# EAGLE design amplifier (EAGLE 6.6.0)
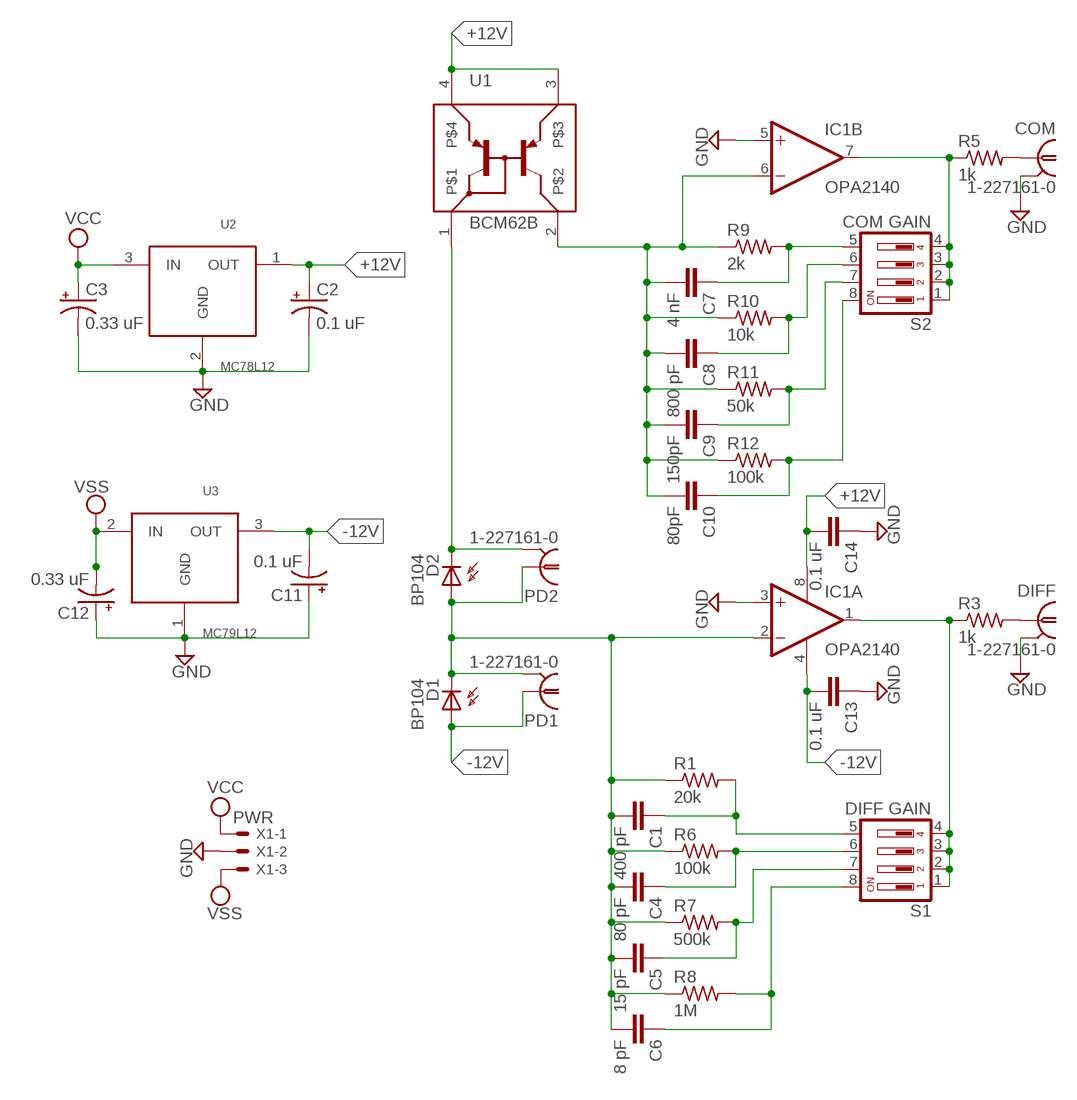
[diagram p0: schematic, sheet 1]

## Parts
C1  400 pF  C-EUC1206K  [C1206K]
C2  0.1 uF  CPOL-USSMCP  [SMC_P]
C3  0.33 uF  CPOL-USSMCP  [SMC_P]
C4  80 pF  C-EUC1206K  [C1206K]
C5  15 pF  C-EUC1206K  [C1206K]
C6  8 pF  C-EUC1206K  [C1206K]
C7  4 nF  C-EUC1206K  [C1206K]
C8  800 pF  C-EUC1206K  [C1206K]
C9  150pF  C-EUC1206K  [C1206K]
C10  80pF  C-EUC1206K  [C1206K]
C11  0.1 uF  CPOL-USSMCP  [SMC_P]
C12  0.33 uF  CPOL-USSMCP  [SMC_P]
C13  0.1 uF  C-EUC1206K  [C1206K]
C14  0.1 uF  C-EUC1206K  [C1206K]
COM  1-227161-0  [AMP_227161]
D1  BP104  [BP104]
D2  BP104  [BP104]
DIFF  1-227161-0  [AMP_227161]
IC1  OPA2140  [SO08]
PD1  1-227161-0  [AMP_227161]
PD2  1-227161-0  [AMP_227161]
R1  20k  R-US_R1206W  [R1206W]
R3  1k  R-US_R1206W  [R1206W]
R5  1k  R-US_R1206W  [R1206W]
R6  100k  R-US_R1206W  [R1206W]
R7  500k  R-US_R1206W  [R1206W]
R8  1M  R-US_R1206W  [R1206W]
R9  2k  R-US_R1206W  [R1206W]
R10  10k  R-US_R1206W  [R1206W]
R11  50k  R-US_R1206W  [R1206W]
R12  100k  R-US_R1206W  [R1206W]
S1  DIFF GAIN  DS04  [DS-04]
S2  COM GAIN  DS04  [DS-04]
U1  BCM62B  [SOT143M]
U2  MC78L12  [TO92-]
U3  MC79L12  [TO92-]
X1  PWR  KK-156-3  [KK-156-3]

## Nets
+12V: C2.+ C14.2 IC1.8(A:V+) U1.3 U1.4 U2.1(OUT)
-12V: C11.- C13.2 D1.A IC1.4(A:V-) PD1.1 U3.3(OUT)
GND: C2.- C3.- C11.+ C12.+ C13.1 C14.1 COM.2 DIFF.2 IC1.3(A:+IN) IC1.5(B:+IN) U2.2(GND) U3.1(GND) X1.2
N$2: C1.1 R1.2 S1.5
N$3: C10.1 R12.2 S2.8
N$5: COM.1 R5.2
N$6: DIFF.1 R3.2
N$8: C1.2 C4.2 C5.2 C6.2 D1.K(C) D2.A IC1.2(A:-IN) PD1.2 PD2.1 R1.1 R6.1 R7.1 R8.1
N$9: D2.K(C) PD2.2 U1.1
N$10: IC1.1(A:OUT) R3.1 S1.1 S1.2 S1.3 S1.4
N$11: C4.1 R6.2 S1.6
N$13: C5.1 R7.2 S1.7
N$14: C6.1 R8.2 S1.8
N$15: IC1.7(B:OUT) R5.1 S2.1 S2.2 S2.3 S2.4
N$16: C9.1 R11.2 S2.7
N$17: C7.1 R9.2 S2.5
N$18: C8.1 R10.2 S2.6
N$20: C7.2 C8.2 C9.2 C10.2 IC1.6(B:-IN) R9.1 R10.1 R11.1 R12.1 U1.2
VCC: C3.+ U2.3(IN) X1.1
VSS: C12.- U3.2(IN) X1.3

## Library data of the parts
C1 C4-C10 C13 C14 = rcl:C-EU: CAPACITOR, European symbol
C2 C3 C11 C12 = rcl:CPOL-US: POLARIZED CAPACITOR, American symbol
COM DIFF PD1 PD2 = con-coax:?227161*: JACK, RIGHT ANGLE, 50 OHM, PCB, BNC; MF: TYCO ELECTRONICS; MPN: 1-227161; OC_FARNELL: unknown; OC_NEWARK: 33B3200
D1 D2 = opto-trans-siemens:BP104: PHOTO DIODE; MF: VISHAY/TELEFUNKEN; MPN: BP104; OC_FARNELL: 1779636; OC_NEWARK: 14M4504
IC1 = Custom parts:OPA2140: Dual Operational Amplifier Low Power, Single-Supply, Rail-To-Rail Operational Amplifier Source: http://focus.ti.com/lit/ds/symlink/opa2345.pdf http://focus.ti.com .. opa241.pdf http://focus.ti.com/lit/ds/symlink/opa2134.pdf
R1 R3 R5-R12 = rcl:R-US_: RESISTOR, American symbol
S1 S2 = switch-dil:DS04: DIL/CODE SWITCH; OC_FARNELL: 9471570; OC_NEWARK: unknown
U1 = Custom parts:BCM62B: BCM61B - PNP/PNP matched double transistor 1.1 General description PNP/PNP matched double transistor in a SOT143B small Surface-Mounted Device (SMD) plastic package. Matched version of BCV62. NPN/NON equivalent: BCM61B 1.2 Features ■ Current gain matching 1.3 Applications ■ Current mirror ■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
U2 = Custom parts:MC78L12: MC78L12 - 100 mA positive +12V voltage resulators The MC78L00A Series of positive voltage regulators are inexpensive, easy–to–use devices suitable for a multitude of applications that require a regulated supply of up to 100 mA. Like their higher powered MC7800 and MC78M00 Series cousins, these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
U3 = Custom parts:MC79L12: MC79L12 - Negative -12V voltage regulator This series of fixed negative-voltage integrated-circuit voltage regulators is designed for a wide range of applications. These include on-card regulation for elimination of noise and distribution problems associated with single-point regulation. In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
X1 = con-molex:KK-156-3: KK 156 HEADER Source: http://www.molex.com/pdm_docs/sd/026604100_sd.pdf; OC_FARNELL: unknown; OC_NEWARK: unknown

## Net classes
0 default: width 0.508 mm, clearance 0.508 mm

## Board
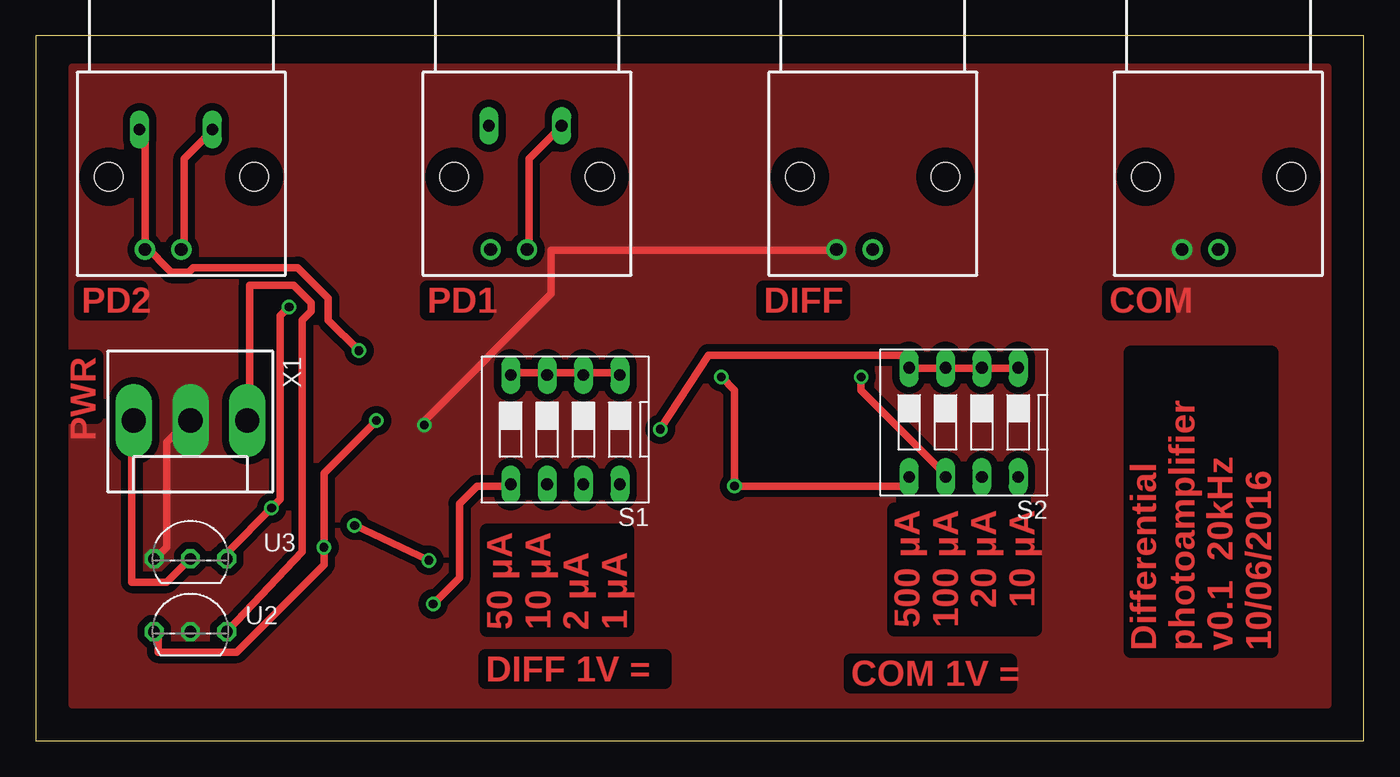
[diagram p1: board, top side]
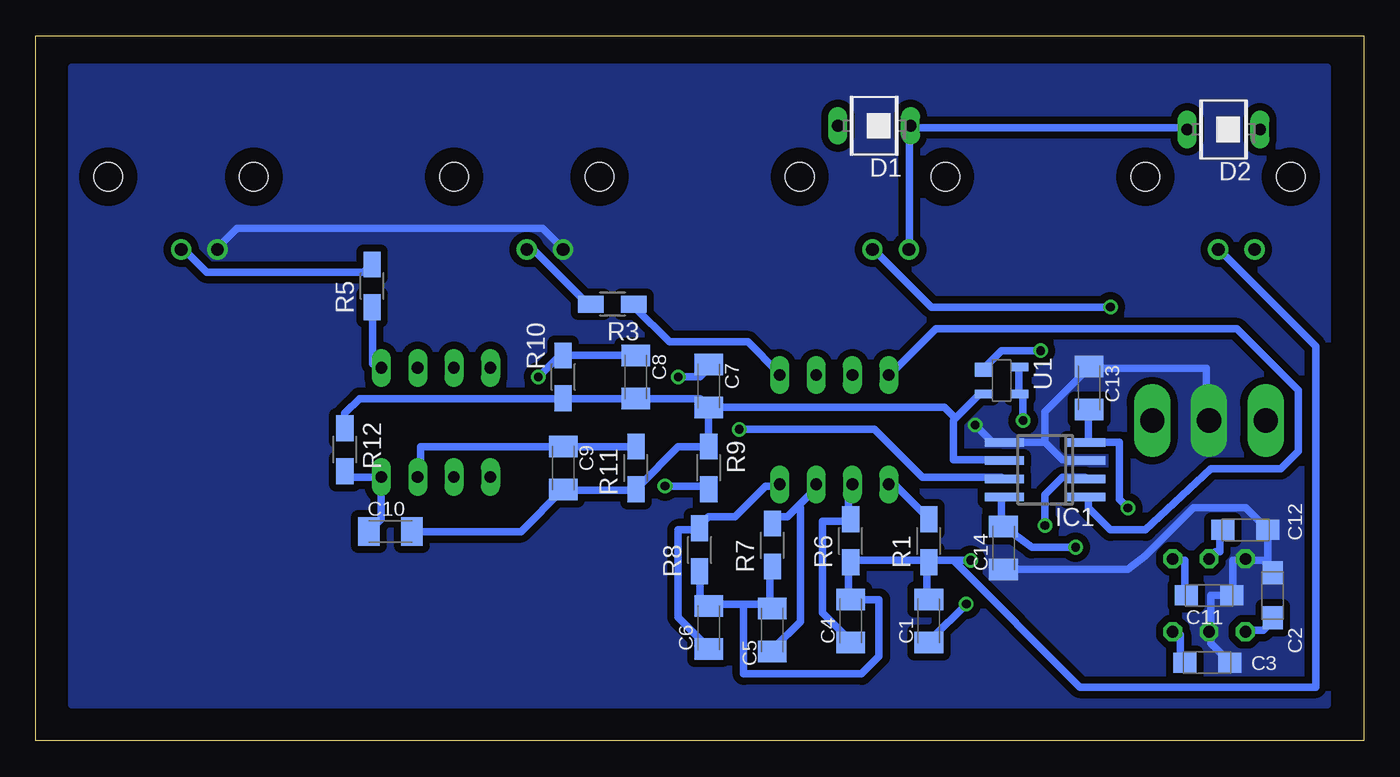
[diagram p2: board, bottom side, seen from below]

Size 92.69 x 49.2 mm. Coordinates in mm from the lower left corner, seen from the top.
Outline: 0,0 92.69,0 92.69,49.2 0,49.2 0,0
Copper layers (1*16): Top 0.035mm / dielectric 1.5mm / Bottom 0.035mm
Design rules "default": minimum track width 10mil, minimum drill 24mil, track to track 8mil, track to pad 8mil, pad to pad 8mil, via to via 8mil, smd to smd 8mil, copper to edge 40mil, drill to drill 8mil, minimum pad ring 10mil, minimum via ring 8mil, stop-mask expansion 4mil, vias tented up to drill 0mil, thermal gap 10mil

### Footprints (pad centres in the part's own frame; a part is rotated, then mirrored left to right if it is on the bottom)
C1206K = smd 1.5 x 2: 1 -1.5,0; 2 1.5,0
SMC_P = smd 1.6 x 1.4: + -1.575,0; - 1.575,0
AMP_227161 = drill 0.9 pad 1.27: 1 0,-5.08; 2 -2.54,-5.08 | hole 2: -5.08,0; 5.08,0
BP104 = drill 0.813 long: A 0,2.54; K 0,-2.54
SO08 = smd 0.6 x 2.708: 1 -1.905,-2.854; 2 -0.635,-2.854; 3 0.635,-2.854; 4 1.905,-2.854; 5 1.905,2.854; 6 0.635,2.854; 7 -0.635,2.854; 8 -1.905,2.854
R1206W = smd 1.8 x 1.2: 1 -1.499,0; 2 1.499,0
DS-04 = drill 0.813 long: 1 -3.81,-3.81; 2 -1.27,-3.81; 3 1.27,-3.81; 4 3.81,-3.81; 5 3.81,3.81; 6 1.27,3.81; 7 -1.27,3.81; 8 -3.81,3.81
SOT143M = smd 1 x 1.208: 1 -0.75,-1.254 | smd 0.6 x 1.208: 2 0.95,-1.254; 3 0.95,1.254; 4 -0.95,1.254
TO92- = drill 0.813 octagon: 1 -2.54,0; 2 0,0; 3 2.54,0
KK-156-3 = drill 1.7 pad 2.184 long: 1 -3.96,0; 2 0,0; 3 3.96,0

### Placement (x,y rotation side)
C1  30.35,8.38 90 bottom
C2  6.35,10.16 90 bottom
C3  10.92,5.46 0 bottom
C4  35.81,8.38 90 bottom
C5  41.27,7.75 90 bottom
C6  45.72,7.9 90 bottom
C7  45.72,24.77 270 bottom
C8  50.8,25.4 270 bottom
C9  55.88,19.05 270 bottom
C10  67.94,14.61 0 bottom
C11  10.79,10.16 180 bottom
C12  8.26,14.73 180 bottom
C13  19.18,24.64 270 bottom
C14  25.15,13.46 90 bottom
COM  82.55,39.37 0 top
D1  34.16,42.93 90 bottom
D2  9.78,42.67 90 bottom
DIFF  58.42,39.37 0 top
IC1  22.23,18.92 90 bottom
PD1  34.29,39.37 0 top
PD2  10.16,39.37 0 top
R1  30.35,13.97 90 bottom
R3  52.45,30.48 180 bottom
R5  69.22,31.75 90 bottom
R6  35.81,13.97 90 bottom
R7  41.27,13.67 90 bottom
R8  46.35,13.34 90 bottom
R9  45.72,19.05 270 bottom
R10  55.88,25.4 90 bottom
R11  50.8,19.05 90 bottom
R12  71.12,20.32 270 bottom
S1  36.96,21.72 180 top
S2  64.77,22.23 180 top
U1  25.27,25.15 270 bottom
U2  10.79,7.62 0 top
U3  10.79,12.7 0 top
X1  10.79,22.35 180 top

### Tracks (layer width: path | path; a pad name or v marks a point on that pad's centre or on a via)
+12V  (via drill 0.61)
  Top 0.508: v23.77,22.35 20.12,18.69 v20.12,13.51 20.12,12.29 14.02,6.2 8.53,6.2 8.53,7.42 U2.1
  Bottom 0.508: IC1.8 25.3,16.87 25.3,15.04 C14.2 23.16,13.51 v20.12,13.51 | U1.4 24.08,26.01 24.08,24.49 U1.3 23.77,24.18 v23.77,22.35 | C2.+ 6.4,8.33 7.01,7.72 8.23,7.72 U2.1
-12V  (via drill 0.61)
  Top 0.508: D1.A 36.58,42.77 34.44,40.64 34.44,34.54 PD1.1 | U3.3 13.41,12.9 13.41,13.21 v16.46,16.26 17.07,16.87 17.07,29.67 v17.68,30.28
  Bottom 0.508: C11.- 12.5,10.16 12.5,12.6 13.11,12.6 U3.3 | C13.2 19.2,22.96 19.2,20.83 IC1.4 17.07,20.83 17.07,16.87 v16.46,16.26 | v17.68,30.28 30.18,30.28 34.14,34.24 PD1.1
GND  (via drill 0.61)
  Top 0.508: X1.2 10.67,22.35 9.14,20.83 9.14,13.51 8.53,12.9 U3.1 | v27.13,22.05 27.13,22.35 35.97,31.19 35.97,34.24 55.78,34.24 DIFF.2
  Bottom 0.508: DIFF.2 56.08,34.54 57.3,35.76 78.64,35.76 79.86,34.54 COM.2 | 22.25,20.83 22.25,22.96 19.2,26.01 C13.1 18.9,26.01 10.97,26.01 10.97,22.35 X1.2 | 22.25,20.83 IC1.5 25.91,20.83 v27.13,22.05 | 22.25,20.83 21.03,19.61 19.51,19.61 IC1.3 | C3.- 9.45,5.59 10.67,6.81 10.67,7.42 U2.2 10.67,7.72 10.67,10.16 C11.+ 9.14,10.16 9.14,12.6 8.53,12.6 U3.1 8.23,12.6 7.01,12.6 6.86,12.45 | 6.86,12.45 6.4,11.99 C2.- | 6.71,14.73 6.71,12.6 6.86,12.45 | 6.71,14.73 8.23,16.26 11.89,16.26 15.24,12.9 16.46,11.96 24.99,11.99 C14.1 | 6.71,14.73 C12.+
  pour Bottom (no thermals): 2.54,46.99 2.54,2.54 90.17,2.54 90.17,46.99
  pour Top (no thermals): 2.54,46.99 2.54,2.54 90.17,2.54 90.17,46.99
N$2  (via drill 0.61)
  Top 0.508: v27.74,9.55 29.57,11.38 29.57,16.56 30.79,17.78 32.92,17.78 S1.5
  Bottom 0.508: R1.2 30.48,15.65 32.61,17.78 32.92,17.78 S1.5 | v27.74,9.55 30.18,7.11 C1.1
N$3
  Bottom 0.508: R12.2 70.71,18.42 S2.8 68.58,15.47 C10.1
N$5
  Bottom 0.508: R5.2 69.49,33.02 69.8,32.72 80.77,32.72 82.3,34.24 COM.1
N$6
  Bottom 0.508: R3.2 54.25,30.58 57.91,34.24 58.22,34.24 DIFF.1
N$8  (via drill 0.61)
  Top 0.508: D2.A 12.19,42.47 10.36,40.64 10.36,34.54 PD2.1 | v27.43,12.6 v22.25,15.04
  Bottom 0.508: PD1.2 31.7,34.54 31.7,42.77 D1.K 31.39,42.77 12.5,42.77 D2.A | 45.72,9.55 46.33,9.55 46.33,11.68 R8.1 | 41.45,9.55 41.45,12.29 R7.1 | 41.45,9.55 43.28,9.55 | 43.28,9.55 45.72,9.55 | 45.72,9.55 C6.2 | 41.45,9.55 C5.2 | R1.1 30.48,12.29 30.48,10.16 C1.2 | 28.65,12.6 30.18,12.6 R1.1 | 28.65,12.6 v27.43,12.6 | R1.1 30.48,12.6 35.66,12.6 R6.1 35.97,12.29 35.97,10.16 C4.2 35.66,9.86 33.83,9.86 33.83,5.89 35.05,4.67 43.28,4.67 43.28,9.55 | 28.65,12.6 19.81,3.76 3.35,3.76 3.35,27.53 10.06,34.24 PD2.1 | v22.25,15.04 22.25,17.17 21.03,18.39 19.47,18.39 IC1.2
N$9  (via drill 0.61)
  Top 0.508: v22.55,27.23 20.42,29.36 20.42,30.89 18.29,33.02 10.97,33.02 10.67,32.72 9.45,32.72 7.62,34.54 | 7.62,34.54 7.62,42.16 7.32,42.47 D2.K | 7.62,34.54 PD2.2
  Bottom 0.508: v22.55,27.23 25.3,27.23 26.52,26.01 U1.1
N$10
  Top 0.508: S1.1 40.54,25.7 38.41,25.7 S1.2 38.1,25.7 35.97,25.7 S1.3 35.66,25.7 33.22,25.7 S1.4
  Bottom 0.508: R3.1 50.9,30.28 48.46,27.84 42.98,27.84 40.84,25.7 S1.1 | S1.4 32.92,25.7 29.87,28.75 8.84,28.75 4.57,24.49 4.57,20.22 5.79,19 10.67,19 15.24,14.73 17.68,14.73 19.2,16.26 19.2,16.85 IC1.1
N$11
  Bottom 0.508: S1.6 35.97,17.78 35.97,15.65 R6.2 35.97,15.34 37.8,15.34 37.8,8.94 35.97,7.11 C4.1
N$13
  Bottom 0.508: 39.47,16.41 38.1,17.78 S1.7 | 39.47,16.41 40.23,15.65 41.15,15.65 R7.2 | C5.1 41.15,6.5 39.32,8.33 39.32,16.26 39.47,16.41
N$14
  Bottom 0.508: S1.8 40.84,17.78 41.76,17.78 43.89,15.65 45.72,15.65 46.33,15.04 R8.2 46.63,14.73 47.85,14.73 47.85,8.64 45.72,6.5 C6.1
N$15  (via drill 0.61)
  Top 0.508: v43.59,21.74 46.94,26.92 60.96,26.92 S2.4 60.96,26.01 63.4,26.01 S2.3 63.7,26.01 65.84,26.01 S2.2 66.14,26.01 68.58,26.01 S2.1
  Bottom 0.508: R5.1 69.19,29.97 69.19,26.31 68.58,26.31 S2.1 | v43.59,21.74 34.14,21.74 30.79,18.39 25.3,18.39 IC1.7
N$16
  Bottom 0.508: R11.2 50.9,20.52 55.78,20.52 C9.1 56.08,20.52 65.84,20.52 65.84,18.69 S2.7
N$17  (via drill 0.61)
  Top 0.508: S2.5 60.96,17.78 v48.77,17.78 48.77,24.49 v47.85,25.4
  Bottom 0.508: v48.77,17.78 45.72,17.78 R9.2 | v47.85,25.4 46.33,25.4 45.72,26.01 C7.1
N$18  (via drill 0.61)
  Top 0.508: v57.61,25.4 57.61,24.49 63.4,18.69 S2.6
  Bottom 0.508: C8.1 50.9,26.92 55.78,26.92 R10.2 56.08,26.62 56.39,26.62 v57.61,25.4
N$20
  Bottom 0.508: 28.5,22.5 28.65,22.35 28.65,19.61 25.3,19.61 IC1.6 | 28.5,22.5 26.82,24.18 U1.2 | C7.2 46.33,23.88 50.6,23.88 C8.2 50.9,23.88 55.78,23.88 R10.1 56.08,23.88 70.1,23.88 71.12,22.86 R12.1 | 28.5,22.5 29.26,23.27 C7.2 | C7.2 R9.1 45.72,20.52 47.85,20.52 50.6,17.78 R11.1 50.9,17.48 55.78,17.48 C9.2 58.83,14.61 C10.2
VCC
  Top 0.508: U2.3 13.41,7.72 18.59,13.21 18.59,29.36 19.2,29.97 19.2,30.58 17.98,31.8 14.94,31.8 14.94,22.35 X1.1
  Bottom 0.508: C3.+ 12.8,5.59 12.8,7.42 13.11,7.42 U2.3
VSS
  Top 0.508: U3.2 10.67,12.6 9.14,11.07 6.71,11.07 6.71,22.35 X1.3
  Bottom 0.508: 9.75,14.73 C12.- 10.06,14.73 10.06,13.21 10.36,13.21 10.67,12.9 U3.2

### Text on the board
Top: 500 μA / 100 μA / 20 μA / 10 μA | 50 μA / 10 μA / 2 μA / 1 μA | Differential / photoamplifier / v0.1 20kHz / 10/06/2016 | DIFF 1V = | COM 1V =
